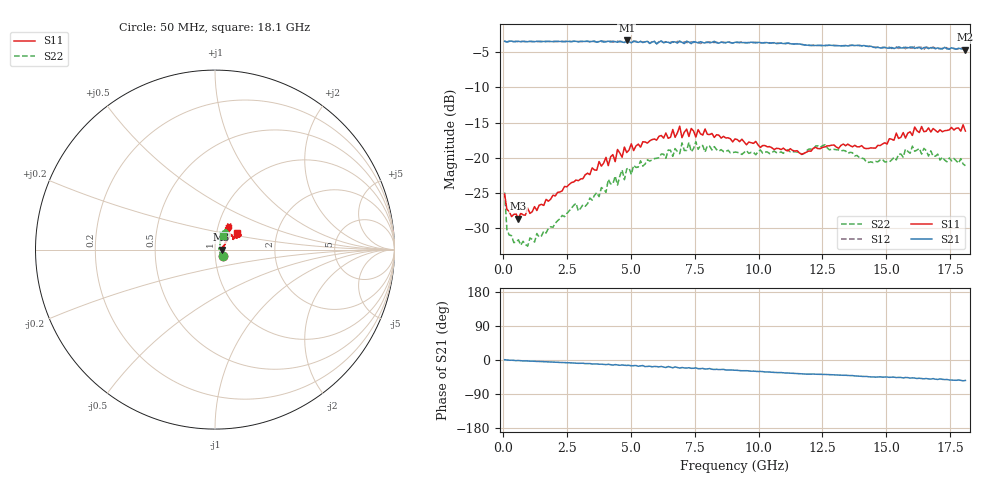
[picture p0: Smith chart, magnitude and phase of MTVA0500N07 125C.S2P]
! Network Analyzer HP8720D.06.14 Serial No. US36140669
!  5 Jul 2005  09:09:10
! Frequency  S11  S21  S12  S22
# HZ  S  DB R 50
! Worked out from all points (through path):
!   201 points, 50 MHz to 18.1 GHz, reference 50 ohm
!   highest |S21| = -3.32 dB at 4.833 GHz (marker M1); lowest = -4.6 dB at 18.1 GHz (marker M2)
!   group delay of S21, straight-line fit = 8.44 ps
!   lowest |S11| = -28.6 dB at 591.5 MHz (marker M3), VSWR 1.08, Z = 53.8 + j0.0286 ohm
!   |S11| at or under -10 dB: start of sweep to end of sweep
!   |S22| runs from -32.6 to -17.7 dB; largest |S21 - S12| = 0.027
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5e7  -25.17 -37.1  -3.43 0.8  -3.45 0.9  -24.93 -42.1
1.4025e8  -27.35 -21.7  -3.54 0.0  -3.51 -0.1  -30.22 -29.6
5.915e8  -28.65 0.4  -3.44 -1.2  -3.49 -1.4  -31.66 2.2
9.525e8  -27.16 8.2  -3.50 -2.6  -3.44 -2.7  -32.57 11.7
3.1185e9  -22.96 35.8  -3.45 -8.5  -3.49 -8.8  -26.67 53.8
4.021e9  -19.94 43.6  -3.50 -12.2  -3.48 -11.4  -24.92 57.3
4.11125e9  -21.12 44.0  -3.42 -11.3  -3.51 -12.2  -23.06 58.2
4.47225e9  -18.82 42.5  -3.58 -13.0  -3.42 -12.6  -23.87 64.5
4.65275e9  -19.92 43.6  -3.54 -13.0  -3.46 -14.1  -21.72 65.4
4.743e9  -18.48 47.6  -3.61 -13.9  -3.52 -13.3  -23.11 61.4
4.83325e9  -19.26 52.8  -3.32 -14.3  -3.49 -14.5  -21.60 55.8
6.09675e9  -16.95 53.3  -3.57 -18.2  -3.48 -18.1  -19.98 60.1
6.7285e9  -17.09 59.9  -3.53 -18.3  -3.75 -18.9  -18.69 57.0
6.909e9  -15.51 58.6  -3.41 -21.4  -3.48 -20.0  -19.42 57.4
6.99925e9  -17.14 58.3  -3.60 -19.9  -3.74 -21.4  -17.90 59.0
7.36025e9  -15.83 54.9  -3.77 -22.0  -3.52 -21.4  -19.15 62.5
7.54075e9  -17.06 57.0  -3.55 -20.9  -3.47 -23.2  -17.71 61.3
9.075e9  -17.32 61.9  -3.59 -27.0  -3.57 -27.1  -19.19 50.3
1.21435e10  -18.64 49.4  -4.03 -37.1  -3.99 -37.3  -18.75 61.9
1.512175e10  -17.29 31.3  -4.41 -45.8  -4.28 -45.4  -20.58 70.7
1.602425e10  -16.82 30.1  -4.25 -47.0  -4.41 -48.9  -18.34 58.5
1.81e10  -16.20 37.8  -4.64 -54.0  -4.76 -54.8  -21.13 58.4
